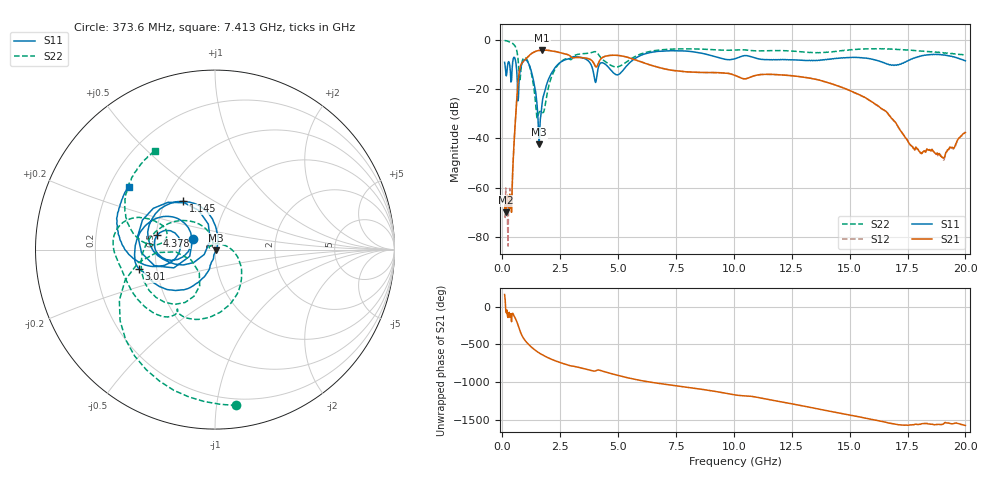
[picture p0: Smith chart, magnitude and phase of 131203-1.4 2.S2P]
!  2-Port S-parameters saved by WinCal
! VAR MeasName=S-Parameters (CALIBRATED_DATA) read from VNA (N5244A)
! VAR MeasDate=4/4/2013 3:56:11 PM
! VAR NAME=131203-1.4 2
! VAR FILENAME=131203-1.4 2.S2P
! VAR DATE=4/4/2013 3:56:12 PM
! VAR PHYS_PORTS=1,2
# Hz S MA R 50
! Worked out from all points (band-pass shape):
!   801 points, 100 MHz to 20 GHz, reference 50 ohm
!   highest |S21| = -4.30 dB at 1.717 GHz (marker M1); lowest = -70.0 dB at 149.8 MHz (marker M2)
!   |S21| within 3 dB of the highest: 1.072 GHz to 3.011 GHz (1.939 GHz wide, 95 % of centre); 4.321 GHz to 5.452 GHz (1.13 GHz wide, 23.1 % of centre)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
!   lowest |S11| = -42.5 dB at 1.593 GHz (marker M3), VSWR 1.02, Z = 50.6 - j0.404 ohm
!   |S11| at or under -10 dB: 1.151 GHz to 2.411 GHz (1.261 GHz wide, 70.8 % of centre); 4.449 GHz to 5.434 GHz (985.4 MHz wide, 19.9 % of centre); 16.68 GHz to 17.16 GHz (480 MHz wide, 2.84 % of centre)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
!   |S22| runs from -31.8 to -0.4 dB; largest |S21 - S12| = 0.0033
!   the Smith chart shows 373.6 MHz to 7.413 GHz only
!   S11 on the Smith chart (normalised r, x): 373.6 MHz: 0.77, +0.10; 1.145 GHz: 0.62, +0.37; 3.01 GHz: 0.40, -0.11; 4.378 GHz: 0.51, +0.09; 7.413 GHz: 0.28, +0.30
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1e8  0.3461 153.0  0.0003859 161.3  0.0006311 80.3  0.96 -22.4
1.4975e8  0.2217 151.2  0.0003153 -50.1  0.0009883 11.8  0.9489 -33.1
3.73625e8  0.138 153.6  0.0006961 -91.4  0.0004655 -118.4  0.8766 -82.2
5.72625e8  0.3715 134.8  0.02587 -160.7  0.02603 -160.5  0.7069 -134.8
7.21875e8  0.1397 -148.7  0.2037 78.5  0.2042 78.6  0.2189 -176.7
8.71125e8  0.3435 -178.6  0.345 -34.3  0.3458 -34.2  0.3783 -126.2
1.14475e9  0.3213 123.2  0.4681 -141.9  0.4692 -141.8  0.3221 157.0
1.5925e9  0.00752 -32.0  0.6018 107.9  0.6035 107.9  0.03396 162.4
1.716875e9  0.0497 -99.2  0.6096 85.3  0.611 85.2  0.03335 127.9
2.23925e9  0.2528 -123.2  0.5799 10.0  0.5815 10.0  0.2308 -51.0
3.010375e9  0.438 -165.8  0.4316 -65.9  0.4326 -65.9  0.4094 -121.0
3.43325e9  0.4314 169.0  0.4299 -92.9  0.4308 -92.9  0.5152 -150.6
4.005375e9  0.1427 154.9  0.2953 -131.5  0.2959 -131.5  0.5699 174.8
4.3785e9  0.3318 166.3  0.4464 -137.3  0.4483 -137.5  0.3779 154.7
5.52275e9  0.3468 -164.2  0.421 131.5  0.4224 131.2  0.3976 174.2
6.741625e9  0.5774 160.3  0.2737 65.4  0.2747 65.2  0.6118 139.6
7.41325e9  0.5952 143.9  0.2357 37.6  0.2359 37.2  0.6438 121.5
1.005e10  0.4103 116.0  0.1882 -87.8  0.1886 -88.2  0.6142 71.3
1.338325e10  0.3766 94.0  0.1619 102.3  0.1617 101.7  0.5457 21.5
1.669162e10  0.3128 69.9  0.02987 -100.0  0.02956 -100.7  0.6481 -39.7
1.9005e10  0.4937 55.2  0.004141 -119.0  0.004084 -118.4  0.5415 -102.1
2e10  0.3719 36.3  0.01308 -132.2  0.01342 -131.8  0.4892 -128.5
